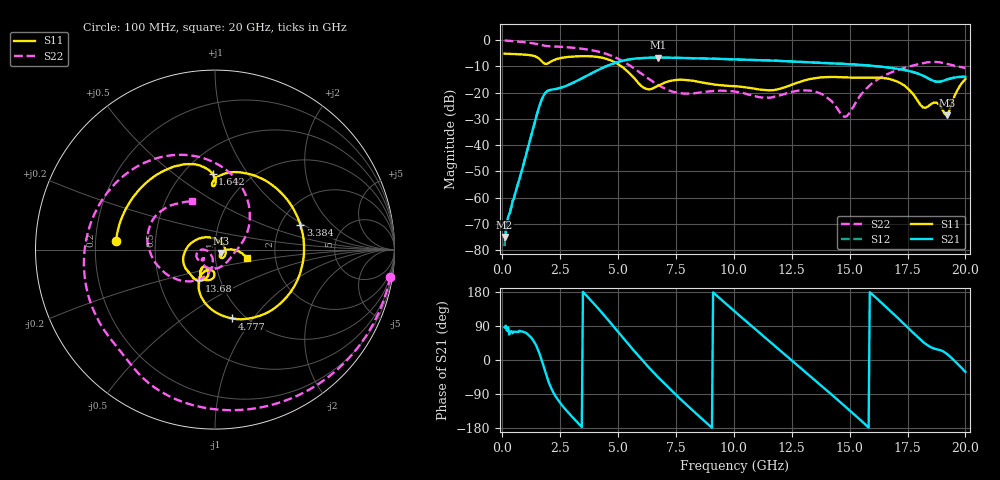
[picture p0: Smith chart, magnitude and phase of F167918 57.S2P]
!  2-Port S-parameters saved by WinCal
! VAR MeasName=S-Parameters (CALIBRATED_DATA) read from VNA (N5242A)
! VAR MeasDate=2016-11-22 10:27:37
! VAR NAME=F167918 57
! VAR FILENAME=F167918 57.S2P
! VAR DATE=2016-11-22 10:27:37
! VAR PHYS_PORTS=1,2
# Hz S DB R 50
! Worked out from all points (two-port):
!   401 points, 100 MHz to 20 GHz, reference 50 ohm
!   highest |S21| = -6.61 dB at 6.717 GHz (marker M1); lowest = -75.0 dB at 100 MHz (marker M2)
!   |S21| within 3 dB of the highest: 4.575 GHz to 15.81 GHz (11.23 GHz wide, 110 % of centre)
!   lowest |S11| = -28.6 dB at 19.2 GHz (marker M3), VSWR 1.08, Z = 53.3 - j2.03 ohm
!   |S11| at or under -10 dB: 5.148 GHz to end of sweep
!   |S22| runs from -29.2 to -0.1 dB; largest |S21 - S12| = 0.0046
!   S11 on the Smith chart (normalised r, x): 100 MHz: 0.29, +0.04; 1.642 GHz: 0.68, +0.70; 3.384 GHz: 2.57, +0.94; 4.777 GHz: 0.88, -0.80; 13.68 GHz: 0.79, -0.28; 20 GHz: 1.42, -0.13
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1e8  -5.14 175.0  -74.98 86.0  -78.44 60.4  -0.10 -8.8
8.4625e8  -5.42 138.0  -49.63 75.1  -49.54 76.8  -0.67 -67.2
1.64225e9  -7.46 91.8  -24.05 10.6  -24.04 10.6  -1.73 -119.4
2.53775e9  -6.78 67.9  -18.07 -116.4  -18.07 -116.5  -2.51 -161.6
3.3835e9  -6.09 16.2  -14.79 -173.7  -14.78 -173.4  -3.18 159.6
3.43325e9  -6.09 13.0  -14.55 -176.8  -14.55 -176.7  -3.24 157.3
4.7765e9  -8.06 -75.8  -8.94 90.7  -8.89 90.7  -6.16 92.1
5.82125e9  -15.77 -119.1  -6.92 14.8  -6.91 14.7  -11.55 42.9
6.71675e9  -17.41 -91.2  -6.61 -44.7  -6.61 -44.6  -16.98 9.3
6.7665e9  -17.19 -91.2  -6.62 -47.7  -6.62 -47.7  -17.25 7.3
7.61225e9  -15.06 -105.4  -6.73 -98.4  -6.73 -98.3  -20.07 -25.0
8.60725e9  -16.08 -122.0  -6.94 -154.4  -6.91 -154.5  -19.84 -72.5
1.005e10  -17.53 -125.2  -7.29 127.5  -7.29 127.6  -19.59 -129.8
1.09455e10  -18.56 -124.7  -7.57 80.4  -7.55 80.4  -21.35 -144.3
1.19405e10  -18.61 -109.5  -7.90 28.2  -7.87 28.1  -21.06 -138.9
1.338325e10  -14.66 -112.4  -8.47 -47.5  -8.42 -47.3  -19.35 -164.1
1.368175e10  -14.27 -117.1  -8.61 -63.0  -8.55 -63.0  -20.07 -171.7
1.4826e10  -14.17 -131.9  -9.11 -123.6  -9.02 -123.9  -29.05 -140.2
1.67165e10  -14.80 -166.0  -10.42 131.8  -10.49 131.5  -12.57 -131.1
1.83085e10  -25.58 29.0  -14.16 41.0  -14.10 41.2  -8.52 175.3
1.9204e10  -28.61 -30.9  -14.96 15.9  -14.93 16.1  -9.03 137.3
2e10  -14.81 -14.4  -13.96 -31.3  -13.90 -31.1  -10.57 115.1
